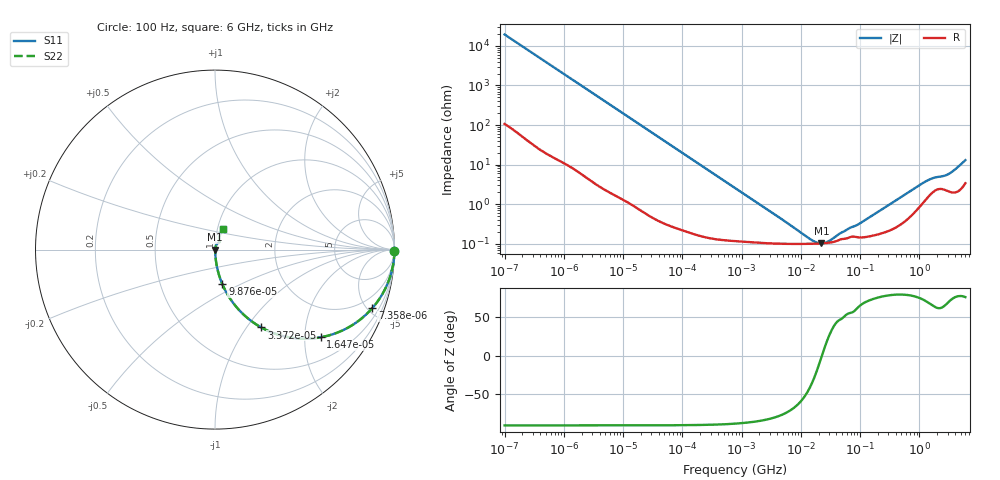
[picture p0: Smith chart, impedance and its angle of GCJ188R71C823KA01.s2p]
!Murata Part Number: GCJ188R71C823KA01
!These Parameters are Measured in Series Mode Connection
!Data Generated on Mar 13, 2026
!  o--ll--o
!Port1  Port2
!  o------o
!Operation Temp=25[degC], DC Bias Voltage=0[V]
!Freq. Start=100[Hz] Stop=6[GHz] 401[Steps]
# Hz S RI R 50
!Freq.(Hz) S11(Real) S11(Imag) S21(Real) S21(Imag) S12(Real) S12(Imag) S22(Real) S22(Imag)
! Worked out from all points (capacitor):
!   401 points, 100 Hz to 6 GHz, reference 50 ohm
!   read as one part in series: C = 81.9 nF near 109 Hz
!   lowest |Z| = 102 mohm at 22.26 MHz (marker M1)
!   series resonance near 22.76 MHz, so ESL is about 600 pH
!   S11 on the Smith chart (normalised r, x): 100 Hz: open; 7.358 kHz: 1.03, -5.35; 16.47 kHz: 1.02, -2.40; 33.72 kHz: 1.01, -1.17; 98.76 kHz: 1.00, -0.40; 6 GHz: 1.07, +0.25
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100  0.9999 -0.00515  5.49e-05 0.00515  5.49e-05 0.00515  0.9999 -0.00515
627  0.9988 -0.0321  0.00119 0.0321  0.00119 0.0321  0.9988 -0.0321
2008  0.989 -0.1013  0.011 0.1013  0.011 0.1013  0.989 -0.1013
4299  0.9532 -0.2083  0.0468 0.2083  0.0468 0.2083  0.9532 -0.2083
7358  0.8758 -0.3267  0.1242 0.3267  0.1242 0.3267  0.8758 -0.3267
11009  0.7608 -0.4233  0.2392 0.4233  0.2392 0.4233  0.7608 -0.4233
16473  0.5892 -0.4886  0.4108 0.4886  0.4108 0.4886  0.5892 -0.4886
23569  0.4138 -0.489  0.5862 0.489  0.5862 0.489  0.4138 -0.489
33721  0.258 -0.4339  0.742 0.4339  0.742 0.4339  0.258 -0.4339
40335  0.1962 -0.3934  0.8038 0.3934  0.8038 0.3934  0.1962 -0.3934
60352  0.0996 -0.2951  0.9004 0.2951  0.9004 0.2951  0.0996 -0.2951
98762  0.0409 -0.1926  0.9591 0.1926  0.9591 0.1926  0.0409 -0.1926
241822  0.00819 -0.0817  0.9918 0.0817  0.9918 0.0817  0.00819 -0.0817
774597  0.00183 -0.0257  0.9982 0.0257  0.9982 0.0257  0.00183 -0.0257
1.555665e7  0.001 -0.000694  0.999 0.000694  0.999 0.000694  0.001 -0.000694
2.225763e7  0.00102 -3.97e-05  0.999 3.97e-05  0.999 3.97e-05  0.00102 -3.97e-05
3.045065e7  0.00106 0.00053  0.9989 -0.00053  0.9989 -0.00053  0.00106 0.00053
9.753859e7  0.00145 0.00287  0.9986 -0.00287  0.9986 -0.00287  0.00145 0.00287
3.124326e8  0.00223 0.00947  0.9978 -0.00947  0.9978 -0.00947  0.00223 0.00947
1.309207e9  0.0145 0.0349  0.9855 -0.0349  0.9855 -0.0349  0.0145 0.0349
3.205649e9  0.0232 0.053  0.9768 -0.053  0.9768 -0.053  0.0232 0.053
6e9  0.0467 0.1155  0.9533 -0.1155  0.9533 -0.1155  0.0467 0.1155
